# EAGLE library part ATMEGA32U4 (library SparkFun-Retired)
Atmel 44-pin 8-bit Microcontroller with 32KBytes of ISP Flash and USB Controller ----- Please use the QFN-44-NOPAD_1:1 package for the footprint of all boards using a 32U4. Route traces directly away from the pads as much as possible.
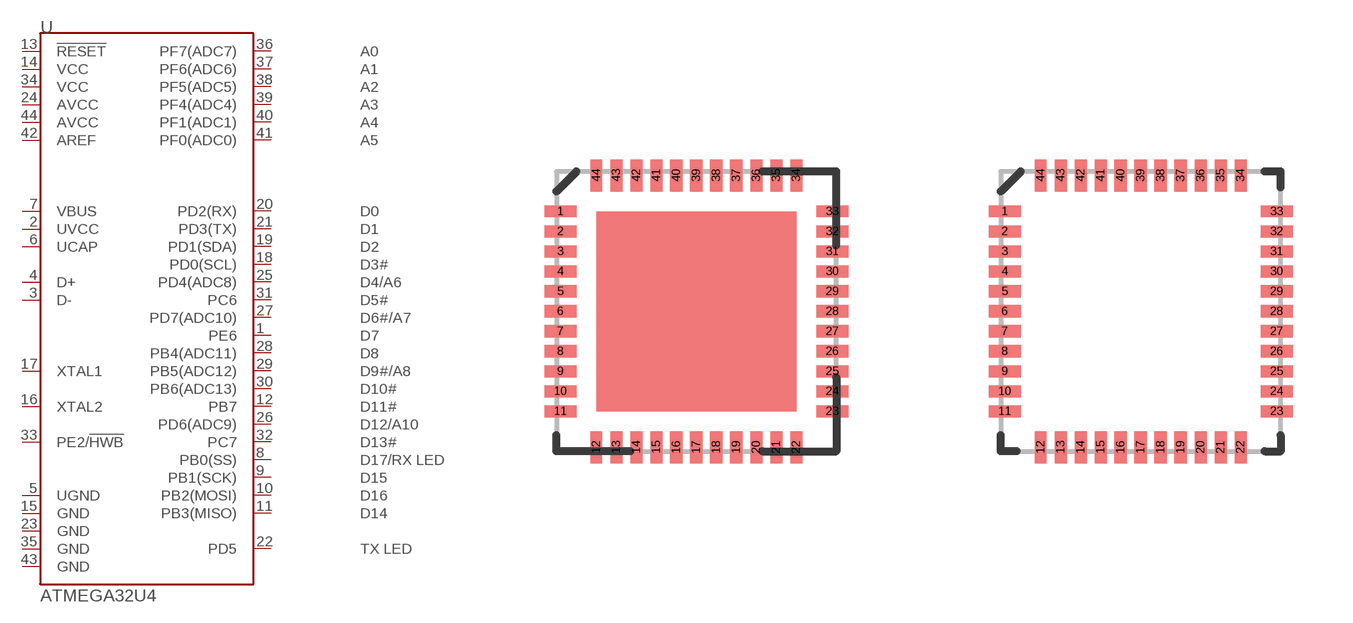
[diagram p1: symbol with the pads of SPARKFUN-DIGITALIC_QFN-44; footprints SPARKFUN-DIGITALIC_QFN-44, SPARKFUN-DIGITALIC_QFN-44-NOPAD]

Designator prefix -

## ATMEGA32U4QFN  [SPARKFUN-DIGITALIC_QFN-44]
1  PE6
2  UVCC
3  D-
4  D+
5  UGND
6  UCAP
7  VBUS
8  PB0(SS)
9  PB1(SCK)
10  PB2(MOSI)
11  PB3(MISO)
12  PB7
13  !RESET
14  VCC
15  GND
16  XTAL2
17  XTAL1
18  PD0(SCL)
19  PD1(SDA)
20  PD2(RX)
21  PD3(TX)
22  PD5
23  GND
24  AVCC
25  PD4(ADC8)
26  PD6(ADC9)
27  PD7(ADC10)
28  PB4(ADC11)
29  PB5(ADC12)
30  PB6(ADC13)
31  PC6
32  PC7
33  PE2/!HWB
34  VCC
35  GND
36  PF7(ADC7)
37  PF6(ADC6)
38  PF5(ADC5)
39  PF4(ADC4)
40  PF1(ADC1)
41  PF0(ADC0)
42  AREF
43  GND
44  AVCC

## ATMEGA32U4QFN2  [SPARKFUN-DIGITALIC_QFN-44-NOPAD]
Pads as for SPARKFUN-DIGITALIC_QFN-44

## ATMEGA32U4TQFP (PROD_ID: IC-11161)  [SPARKFUN-DIGITALIC_TQFP44]
Pads as for SPARKFUN-DIGITALIC_QFN-44

## ATMEGA32U4QFN_1:1  [QFN-44-NOPAD_1:1]
Pads as for SPARKFUN-DIGITALIC_QFN-44

## Footprint SPARKFUN-DIGITALIC_QFN-44 (pad centres in mm)
smd 0.8 x 0.3: 1 -3.4,2.5; 2 -3.4,2; 3 -3.4,1.5; 4 -3.4,1; 5 -3.4,0.5; 6 -3.4,0; 7 -3.4,-0.5; 8 -3.4,-1; 9 -3.4,-1.5; 10 -3.4,-2; 11 -3.4,-2.5; 23 3.4,-2.5; 24 3.4,-2; 25 3.4,-1.5; 26 3.4,-1; 27 3.4,-0.5; 28 3.4,0; 29 3.4,0.5; 30 3.4,1; 31 3.4,1.5; 32 3.4,2; 33 3.4,2.5
smd 0.3 x 0.8: 12 -2.5,-3.4; 13 -2,-3.4; 14 -1.5,-3.4; 15 -1,-3.4; 16 -0.5,-3.4; 17 0,-3.4; 18 0.5,-3.4; 19 1,-3.4; 20 1.5,-3.4; 21 2,-3.4; 22 2.5,-3.4; 34 2.5,3.4; 35 2,3.4; 36 1.5,3.4; 37 1,3.4; 38 0.5,3.4; 39 0,3.4; 40 -0.5,3.4; 41 -1,3.4; 42 -1.5,3.4; 43 -2,3.4; 44 -2.5,3.4

## Footprint SPARKFUN-DIGITALIC_QFN-44-NOPAD (pad centres in mm)
smd 0.8 x 0.3: 1 -3.4,2.5; 2 -3.4,2; 3 -3.4,1.5; 4 -3.4,1; 5 -3.4,0.5; 6 -3.4,0; 7 -3.4,-0.5; 8 -3.4,-1; 9 -3.4,-1.5; 10 -3.4,-2; 11 -3.4,-2.5; 23 3.4,-2.5; 24 3.4,-2; 25 3.4,-1.5; 26 3.4,-1; 27 3.4,-0.5; 28 3.4,0; 29 3.4,0.5; 30 3.4,1; 31 3.4,1.5; 32 3.4,2; 33 3.4,2.5
smd 0.3 x 0.8: 12 -2.5,-3.4; 13 -2,-3.4; 14 -1.5,-3.4; 15 -1,-3.4; 16 -0.5,-3.4; 17 0,-3.4; 18 0.5,-3.4; 19 1,-3.4; 20 1.5,-3.4; 21 2,-3.4; 22 2.5,-3.4; 34 2.5,3.4; 35 2,3.4; 36 1.5,3.4; 37 1,3.4; 38 0.5,3.4; 39 0,3.4; 40 -0.5,3.4; 41 -1,3.4; 42 -1.5,3.4; 43 -2,3.4; 44 -2.5,3.4

## Footprint SPARKFUN-DIGITALIC_TQFP44 (pad centres in mm)
smd 1.5 x 0.5: 1 -5.8,4; 2 -5.8,3.2; 3 -5.8,2.4; 4 -5.8,1.6; 5 -5.8,0.8; 6 -5.8,0; 7 -5.8,-0.8; 8 -5.8,-1.6; 9 -5.8,-2.4; 10 -5.8,-3.2; 11 -5.8,-4; 23 5.8,-4; 24 5.8,-3.2; 25 5.8,-2.4; 26 5.8,-1.6; 27 5.8,-0.8; 28 5.8,0; 29 5.8,0.8; 30 5.8,1.6; 31 5.8,2.4; 32 5.8,3.2; 33 5.8,4
smd 0.5 x 1.5: 12 -4,-5.8; 13 -3.2,-5.8; 14 -2.4,-5.8; 15 -1.6,-5.8; 16 -0.8,-5.8; 17 0,-5.8; 18 0.8,-5.8; 19 1.6,-5.8; 20 2.4,-5.8; 21 3.2,-5.8; 22 4,-5.8; 34 4,5.8; 35 3.2,5.8; 36 2.4,5.8; 37 1.6,5.8; 38 0.8,5.8; 39 0,5.8; 40 -0.8,5.8; 41 -1.6,5.8; 42 -2.4,5.8; 43 -3.2,5.8; 44 -4,5.8

## Footprint QFN-44-NOPAD_1:1 (pad centres in mm)
smd 0.8 x 0.3: 1 -3.337,2.458; 2 -3.337,1.958; 3 -3.337,1.479; 4 -3.337,0.979; 5 -3.337,0.5; 6 -3.337,0; 7 -3.337,-0.5; 8 -3.337,-0.979; 9 -3.337,-1.479; 10 -3.337,-1.958; 11 -3.337,-2.458; 23 3.337,-2.458; 24 3.337,-1.958; 25 3.337,-1.479; 26 3.337,-0.979; 27 3.337,-0.5; 28 3.337,0; 29 3.337,0.5; 30 3.337,0.979; 31 3.337,1.479; 32 3.337,1.958; 33 3.337,2.458
smd 0.3 x 0.8: 12 -2.458,-3.337; 13 -1.958,-3.337; 14 -1.479,-3.337; 15 -0.979,-3.337; 16 -0.5,-3.337; 17 0,-3.337; 18 0.5,-3.337; 19 0.979,-3.337; 20 1.479,-3.337; 21 1.958,-3.337; 22 2.458,-3.337; 34 2.458,3.337; 35 1.958,3.337; 36 1.479,3.337; 37 0.979,3.337; 38 0.5,3.337; 39 0,3.337; 40 -0.5,3.337; 41 -0.979,3.337; 42 -1.479,3.337; 43 -1.958,3.337; 44 -2.458,3.337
